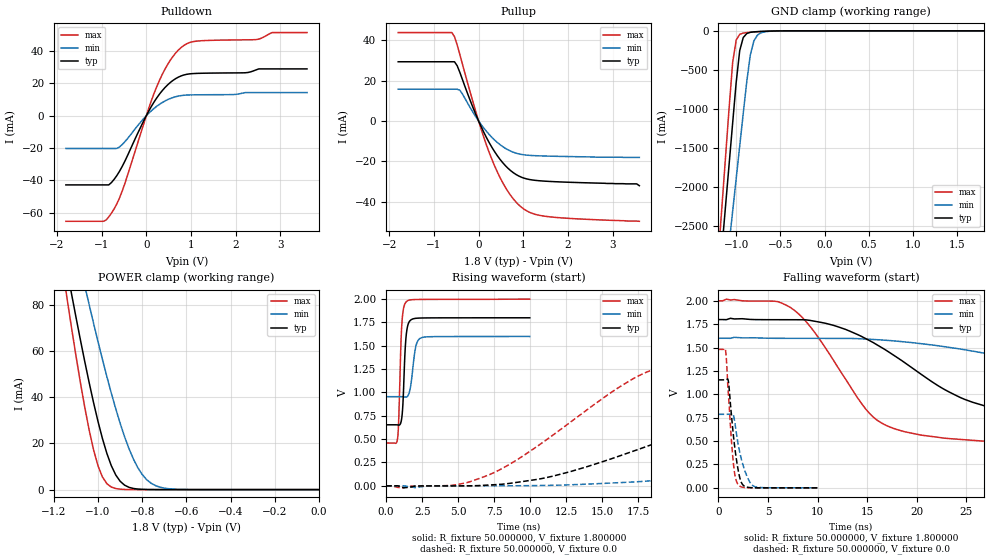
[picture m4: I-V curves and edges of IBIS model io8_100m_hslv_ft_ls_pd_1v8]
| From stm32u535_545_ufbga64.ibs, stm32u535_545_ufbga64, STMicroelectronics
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|   Model io8_100m_hslv_ft_ls_pd_1v8
[Model]  io8_100m_hslv_ft_ls_pd_1v8
Model_type I/O
Polarity   Non-Inverting
Enable   Active-Low
Vinl =   0.540000V
Vinh =   1.260000V
Vmeas =  0.900000V
Cref =   50.000000pF
Rref =   100.000000M
Vref =   0.0V
C_comp   3.235100pF   3.233100pF   3.282800pF
[Temperature Range]   25.000000   0.140000k   -40.000000
[Pullup Reference]   1.800000V   1.600000V   2.000000V
[Pulldown Reference]   0.0V   0.0V   0.0V
[POWER Clamp Reference]   1.800000V   1.600000V   2.000000V
[GND Clamp Reference]   0.0V   0.0V   0.0V
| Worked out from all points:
|   slope of the pulldown table from 0 to 0.27 V, typ, clamps not added: 21.7 ohm
|   slope of the pullup table from 0 to 0.27 V, typ, clamps not added: 22.6 ohm
|   GND clamp passes 1 mA (typ) near -0.51 V on its own axis
|   POWER clamp passes 1 mA (typ) near -0.86 V on its own axis
|   rising waveform, R_fixture 50.000000, V_fixture 1.800000: 20-80 % time 203ps typ, 317ps min, 190ps max; typ from 0.654 V to 1.8 V
|   rising waveform, R_fixture 50.000000, V_fixture 0.0: 20-80 % time 14.5ns typ, 29.3ns min, 8.35ns max; typ from 0 V to 1.15 V
|   falling waveform, R_fixture 50.000000, V_fixture 1.800000: 20-80 % time 11.3ns typ, 24.9ns min, 6.02ns max; typ from 1.8 V to 0.654 V
|   falling waveform, R_fixture 50.000000, V_fixture 0.0: 20-80 % time 732ps typ, 1ns min, 579ps max; typ from 1.15 V to 0 V
[Pulldown]
|Voltage   I(typ)   I(min)   I(max)
-1.8V     -42.74mA   -20.21mA   -65.25mA
-960mV    -42.74mA   -20.21mA   -65.25mA
-780mV    -41.3mA    -20.21mA   -60.25mA
-540mV    -31.39mA   -17.82mA   -46.65mA
0V        0A         -900fA     0A
240mV     11.28mA    6.001mA    18.38mA
480mV     19.17mA    10.02mA    31.83mA
780mV     24.67mA    12.49mA    42.21mA
1.14V     26.24mA    12.99mA    46.23mA
2.46V     28.42mA    14.39mA    47.14mA
2.82V     29mA       14.39mA    51.49mA
3.6V      29mA       14.39mA    51.49mA
[Pullup]
|Voltage   I(typ)   I(min)   I(max)
-1.8V     29.28mA    15.71mA    43.71mA
-600mV    29.28mA    15.71mA    43.71mA
-540mV    29.28mA    15.71mA    41.72mA
-420mV    24.04mA    15.23mA    32.87mA
0V        0A         0A         0A
300mV     -13.1mA    -8.157mA   -19.11mA
600mV     -22.1mA    -13.53mA   -32.82mA
780mV     -25.61mA   -15.48mA   -38.6mA
960mV     -27.82mA   -16.55mA   -42.66mA
1.2V      -29.16mA   -17.08mA   -45.68mA
1.56V     -29.85mA   -17.37mA   -47.3mA
3.6V      -32mA      -18mA      -49.6mA
[GND_clamp]
|Voltage   I(typ)   I(min)   I(max)
-1.8V     -9.707A    -9.942A    -9.774A
-1.2V     -3.309A    -4.006A    -2.865A
-1.16V    -2.777A    -3.584A    -2.239A
-1.12V    -2.246A    -3.162A    -1.614A
-1.04V    -1.186A    -2.319A    -408.7mA
-1V       -663.9mA   -1.898A    -117.8mA
-960mV    -254mA     -1.478A    -45.15mA
-920mV    -86.04mA   -1.06A     -28.6mA
-840mV    -19.13mA   -308.9mA   -18.75mA
-800mV    -13.4mA    -130.8mA   -15.33mA
-720mV    -7.959mA   -25.38mA   -9.395mA
1.8V      45.71uA    33.33uA    56.11uA
[POWER_clamp]
|Voltage   I(typ)   I(min)   I(max)
-1.8V     470.8mA    433.7mA    554.6mA
-1.14V    95.25mA    122.7mA    82.82mA
-1.12V    84.97mA    114mA      70.27mA
-1.06V    55.51mA    88.42mA    35.67mA
-1.04V    46.34mA    80.15mA    25.76mA
-1V       29.51mA    64.13mA    10.3mA
-940mV    10.39mA    41.86mA    1.109mA
-900mV    3.624mA    28.77mA    182.8uA
-840mV    490.7uA    13.24mA    11.35uA
-800mV    116.8uA    6.532mA    1.77uA
-740mV    13.2uA     1.723mA    109.2nA
0V        0A         18.72nA    0A
[Ramp]
| variable   typ   min   max
dV/dt_r  0.69258/14.45285n   0.47157/29.25683n   0.88824/8.34186n
dV/dt_f  0.68753/11.33025n   0.38684/24.87530n   0.92451/6.00658n
R_load = 50.000000
[Rising Waveform]
R_fixture= 50.000000
V_fixture= 1.800000
V_fixture_min= 1.600000
V_fixture_max= 2.000000
|time   V(typ)   V(min)   V(max)
0s        653.5mV    954.5mV    458.4mV
780.8ps   652.7mV    954.4mV    495.1mV
860.9ps   650.1mV    954.5mV    662.6mV
1.081ns   723.3mV    954.4mV    1.711V
1.201ns   1.004V     953.5mV    1.895V
1.401ns   1.624V     950.6mV    1.972V
1.702ns   1.775V     1.068V     1.992V
2.062ns   1.794V     1.494V     1.995V
2.402ns   1.797V     1.583V     1.996V
9.97ns    1.799V     1.599V     1.999V
[Rising Waveform]
R_fixture= 50.000000
V_fixture= 0.0
V_fixture_min= 0.0
V_fixture_max= 0.0
|time   V(typ)   V(min)   V(max)
0s        2.11nV     142.9nV    1.438nV
6.006ns   574.2uV    -347.2uV   53.6mV
11.21ns   90.98mV    4.452mV    502.1mV
18.02ns   417.9mV    49.41mV    1.213V
21.62ns   611.6mV    99.78mV    1.359V
26.83ns   849.9mV    193.2mV    1.434V
40.04ns   1.096V     442.3mV    1.476V
54.45ns   1.142V     631.9mV    1.48V
72.07ns   1.153V     734.9mV    1.48V
199.4ns   1.154V     786.1mV    1.48V
[Falling Waveform]
R_fixture= 50.000000
V_fixture= 1.800000
V_fixture_min= 1.600000
V_fixture_max= 2.000000
|time   V(typ)   V(min)   V(max)
0s        1.799V     1.599V     1.999V
5.606ns   1.798V     1.599V     1.996V
7.608ns   1.798V     1.598V     1.902V
9.61ns    1.783V     1.598V     1.675V
14.81ns   1.597V     1.591V     846.6mV
16.82ns   1.477V     1.578V     671.9mV
26.43ns   889.6mV    1.447V     501.9mV
42.44ns   701.7mV    1.15V      464.1mV
64.06ns   662.4mV    1.019V     458.9mV
199.4ns   653.5mV    954.5mV    458.4mV
[Falling Waveform]
R_fixture= 50.000000
V_fixture= 0.0
V_fixture_min= 0.0
V_fixture_max= 0.0
|time   V(typ)   V(min)   V(max)
0s        1.154V     786.1mV    1.48V
720.7ps   1.154V     786.3mV    1.463V
800.8ps   1.156V     786.3mV    1.366V
1.001ns   1.136V     786.5mV    994.7mV
1.461ns   603.9mV    789.6mV    307.6mV
1.662ns   415.8mV    688.1mV    134.4mV
1.982ns   191.1mV    467.8mV    35.12mV
2.462ns   31.16mV    247.2mV    5.646mV
3.483ns   1.149mV    22.17mV    426.4uV
9.97ns    2.11nV     142.9nV    1.438nV
